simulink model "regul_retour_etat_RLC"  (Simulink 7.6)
settings: Solver=ode23tb  StartTime=0.0  StopTime=0.25  RelTol=1e-3
InitFcn:
  | % valeurs de R, L et C
  | R=3.3;
  | L=100e-3;
  | C=1e-3;
  | 
  | % coefficients du retour d'état
  | f1=-0.1568;
  | f2= -0.6909;
StopFcn:
  | close all, clc
  | load ui.mat
  | 
  | plot(x(1,:),x(2,:),x(1,:),x(3,:),x(1,:),x(4,:),x(1,:),x(5,:))
  | xlabel('temps')
  | title('Régulation de la tension u et du courant i par d''état')
  | grid
undefined symbols (not defined in the file or in its folder): T
libraries: powerlib x8

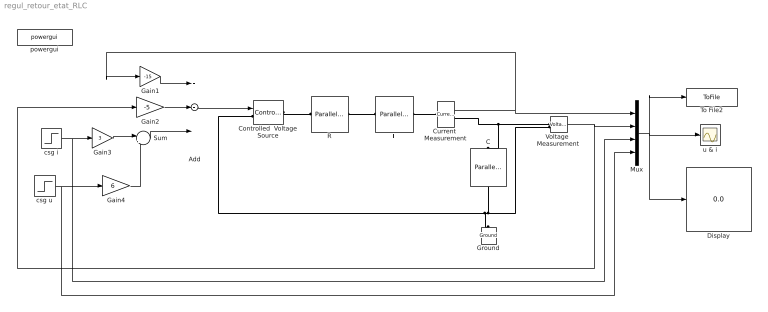
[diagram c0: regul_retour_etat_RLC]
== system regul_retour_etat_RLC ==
  Add : Sum  Inputs=+++
  C : powerlib/Elements/Parallel RLC Branch  DialogController=POWERSYS.PowerSysDialog  PhysicalDomain=powersysdomain  SubClassName=unknown  LeftPortType=p1  RightPortType=p1  LConnTagsString=a  RConnTagsString=__new0  BranchType=C  Resistance=1e-3  Inductance=1e-3  SetiL0=off  InitialCurrent=0  Capacitance=C  Setx0=on  InitialVoltage=0.1  Measurements=None
  Controlled  Voltage Source : powerlib/Electrical Sources/Controlled Voltage Source  DialogController=POWERSYS.PowerSysDialog  SystemSampleTime=-1  Initialize=on  Source_Type=AC  Amplitude=0  Phase=0  Frequency=0  Measurements=None
  Current  Measurement : powerlib/Measurements/Current Measurement  DialogController=POWERSYS.PowerSysDialog  SystemSampleTime=-1  PhasorSimulation=off  OutputType=Complex  PSBequivalent=0
  Display : Display
  Gain1 : Gain  Gain=-15
  Gain2 : Gain  Gain=-5
  Gain3 : Gain  Gain=3
  Gain4 : Gain  Gain=6
  Ground : powerlib/Elements/Ground  DialogController=POWERSYS.PowerSysDialog  PhysicalDomain=powersysdomain  SubClassName=unknown  LeftPortType=p1  RightPortType=p1  LConnTagsString=a
  L : powerlib/Elements/Parallel RLC Branch  DialogController=POWERSYS.PowerSysDialog  PhysicalDomain=powersysdomain  SubClassName=unknown  LeftPortType=p1  RightPortType=p1  LConnTagsString=a  RConnTagsString=__new0  BranchType=L  Resistance=1e-3  Inductance=L  SetiL0=on  InitialCurrent=-0.04  Capacitance=1e-6  Setx0=off  InitialVoltage=0  Measurements=None
  Mux : Mux
  R : powerlib/Elements/Parallel RLC Branch  DialogController=POWERSYS.PowerSysDialog  PhysicalDomain=powersysdomain  SubClassName=unknown  LeftPortType=p1  RightPortType=p1  LConnTagsString=a  RConnTagsString=__new0  BranchType=R  Resistance=R  Inductance=1e-3  SetiL0=off  InitialCurrent=0  Capacitance=1e-6  Setx0=off  InitialVoltage=0  Measurements=None
  Sum : Sum  Inputs=|++
  To File2 : ToFile  Filename=ui  MatrixName=x
  Voltage  Measurement : powerlib/Measurements/Voltage Measurement  DialogController=POWERSYS.PowerSysDialog  SystemSampleTime=-1  PhasorSimulation=off  OutputType=Complex  PSBequivalent=0
  csg i : Step  Time=0  Before=-0.2  After=0  SampleTime=0
  csg u : Step  Time=0.05  After=0.2  SampleTime=0
  powergui : powerlib/powergui  Priority=1  SystemSampleTime=-1  SimulationMode=Continuous  SampleTime=T  frequency=60  SPID=off  DisableSnubberDevices=off  DisableRonSwitches=off  DisableVfSwitches=off  SwTol=0  Interpol=off  frequencyindice=0  echomessages=off  HookPort=off  DisplayEquations=off  FunctionMessages=off  EnableUseOfTLC=off  x0status=blocks  RestoreLinks=warning  ResistiveCurrentMeasurement=off  Ylog=off  Xlog=on  ShowGrid=off  save=off  variable=ZData  ZoomFFT=off  StartTime=0.0  cycles=1  DisplayStyle=1  FreqAxis=off  MaxFrequency=1000  frequencyindicesteady=1  display=off  methode=off
  u & i : Scope
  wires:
  Voltage  Measurement/1 -> Mux/2, Gain2/1
  Current  Measurement/1 -> Mux/1, Gain1/1
  Gain1/1 -> Add/1
  Gain2/1 -> Add/2
  Add/1 -> Controlled  Voltage Source/1
  csg i/1 -> Gain3/1, Mux/3
  csg u/1 -> Gain4/1, Mux/4
  Gain3/1 -> Sum/1
  Sum/1 -> Add/3
  Gain4/1 -> Sum/2
  Mux/1 -> u & i/1, To File2/1, Display/1
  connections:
  R/RConn1 -- L/LConn1
  Voltage  Measurement/LConn1 -- C/LConn1 -- Current  Measurement/RConn1
  C/RConn1 -- Ground/LConn1 -- Controlled  Voltage Source/LConn1 -- Voltage  Measurement/LConn2
  Controlled  Voltage Source/RConn1 -- R/LConn1
  L/RConn1 -- Current  Measurement/LConn1
